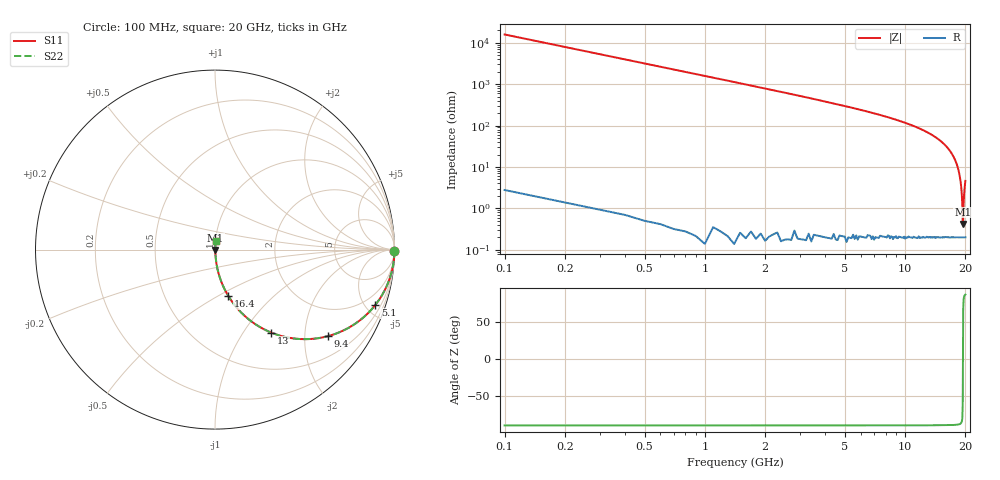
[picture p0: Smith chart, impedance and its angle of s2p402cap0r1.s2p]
! AVX Thin Film Operation		Date: April 2003
! Description: Accu-P® Series, Thin Film, SMD, RF Capacitor
! Part Number: 04021J0R1ABS
! 50 MHz  -  20 GHz
! Serial Measurements
# hz S db R 50
!	S11		S21		S12		S22
!	dB	Phase	dB	Phase	dB	Phase	dB	Phase
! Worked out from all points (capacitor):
!   200 points, 100 MHz to 20 GHz, reference 50 ohm
!   read as one part in series: C = 100 fF near 200 MHz
!   lowest |Z| = 420 mohm at 19.4 GHz (marker M1)
!   series resonance near 19.44 GHz, so ESL is about 670 pH
!   S11 on the Smith chart (normalised r, x): 100 MHz: open; 5.1 GHz: 1.00, -5.81; 9.4 GHz: 1.00, -2.59; 13 GHz: 1.00, -1.35; 16.4 GHz: 1.00, -0.56; 20 GHz: 1.00, +0.09
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1e8  -0.00 -0.4  -44.04 89.6  -44.04 89.6  -0.00 -0.4
2e8  -0.00 -0.7  -38.02 89.3  -38.02 89.3  -0.00 -0.7
4e8  -0.00 -1.4  -31.99 88.5  -31.99 88.5  -0.00 -1.4
1e9  -0.02 -3.6  -24.03 86.4  -24.03 86.4  -0.02 -3.6
3.5e9  -0.22 -12.8  -13.09 77.2  -13.09 77.2  -0.22 -12.8
5.1e9  -0.49 -19.0  -9.75 71.0  -9.75 71.0  -0.49 -19.0
6.8e9  -0.93 -25.9  -7.18 64.0  -7.18 64.0  -0.93 -25.9
9.4e9  -2.03 -37.6  -4.29 52.3  -4.29 52.3  -2.03 -37.6
1.01e10  -2.45 -41.0  -3.67 49.0  -3.67 49.0  -2.45 -41.0
1.3e10  -5.04 -55.8  -1.65 34.0  -1.65 34.0  -5.04 -55.8
1.34e10  -5.54 -57.9  -1.44 31.9  -1.44 31.9  -5.54 -57.9
1.64e10  -11.40 -74.0  -0.34 15.6  -0.34 15.6  -11.40 -74.0
1.67e10  -12.32 -75.5  -0.28 14.0  -0.28 14.0  -12.32 -75.5
1.8e10  -18.05 -81.9  -0.09 7.2  -0.09 7.2  -18.05 -81.9
1.88e10  -25.20 -84.8  -0.03 3.1  -0.03 3.1  -25.20 -84.8
1.92e10  -33.67 -83.3  -0.02 1.2  -0.02 1.2  -33.67 -83.3
1.93e10  -38.20 -80.0  -0.02 0.7  -0.02 0.7  -38.20 -80.0
1.94e10  -47.54 -61.4  -0.02 0.2  -0.02 0.2  -47.54 -61.4
1.95e10  -45.82 66.8  -0.02 -0.3  -0.02 -0.3  -45.82 66.8
1.96e10  -37.58 80.6  -0.02 -0.7  -0.02 -0.7  -37.58 80.6
1.97e10  -33.36 83.4  -0.02 -1.2  -0.02 -1.2  -33.36 83.4
2e10  -26.73 84.9  -0.03 -2.6  -0.03 -2.6  -26.73 84.9
